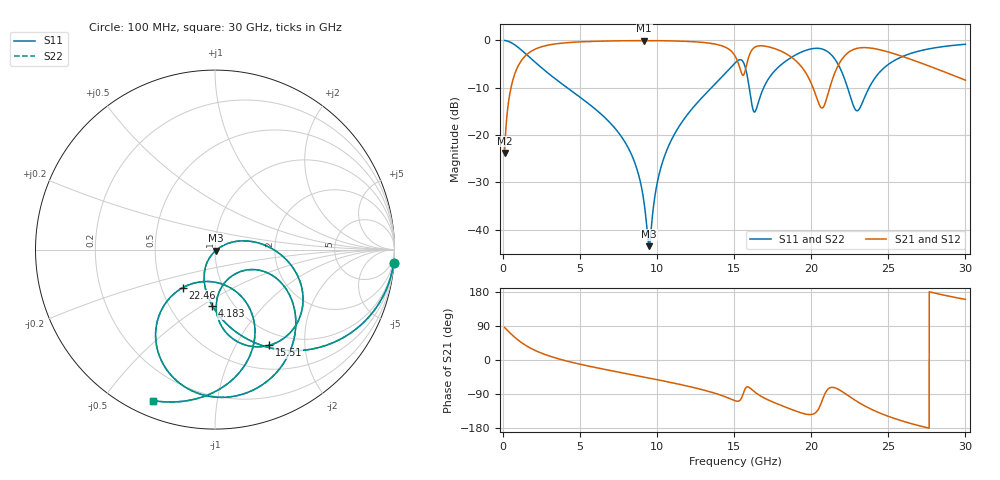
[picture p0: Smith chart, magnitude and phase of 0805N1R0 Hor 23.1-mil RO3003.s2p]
# GHz S MA R 50
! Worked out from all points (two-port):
!   3201 points, 100 MHz to 30 GHz, reference 50 ohm
!   highest |S21| = -0.06 dB at 9.163 GHz (marker M1); lowest = -23.8 dB at 100 MHz (marker M2)
!   |S21| within 3 dB of the highest: 1.516 GHz to 15.01 GHz (13.49 GHz wide, 163 % of centre); 22.23 GHz to 25.6 GHz (3.372 GHz wide, 14.1 % of centre)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
!   lowest |S11| = -43.5 dB at 9.472 GHz (marker M3), VSWR 1.01, Z = 50.4 - j0.519 ohm
!   |S11| at or under -10 dB: 4.151 GHz to 13.53 GHz (9.378 GHz wide, 106 % of centre); 15.97 GHz to 16.91 GHz (937.6 MHz wide, 5.7 % of centre); 22.35 GHz to 23.75 GHz (1.399 GHz wide, 6.07 % of centre)
!   |S22| runs from -43.5 to 0.0 dB; largest |S21 - S12| = 0
!   S11 on the Smith chart (normalised r, x): 100 MHz: 1, -27; 4.183 GHz: 0.80, -0.56; 15.51 GHz: 0.81, -1.39; 22.46 GHz: 0.64, -0.30; 30 GHz: 0.07, -0.67
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0.1  0.9979 -4.2  0.06446 85.8  0.06446 85.8  0.9979 -4.2
0.5017812  0.951 -20.6  0.3086 69.4  0.3086 69.4  0.951 -20.6
1.127813  0.806 -42.1  0.5908 47.9  0.5908 47.9  0.806 -42.1
4.183219  0.3134 -92.7  0.9462 -3.3  0.9462 -3.3  0.3134 -92.7
5.089563  0.244 -101.1  0.9659 -12.0  0.9659 -12.0  0.244 -101.1
7.958094  0.08149 -121.9  0.991 -35.7  0.991 -35.7  0.08149 -121.9
9.163438  0.01855 -115.2  0.9932 -45.2  0.9932 -45.2  0.01855 -115.2
9.471781  0.006665 -50.5  0.993 -47.7  0.993 -47.7  0.006665 -50.5
10.06978  0.03503 25.4  0.9917 -52.5  0.9917 -52.5  0.03503 25.4
13.4055  0.3016 2.6  0.9334 -83.6  0.9334 -83.6  0.3016 2.6
15.05  0.5766 -31.9  0.6847 -107.4  0.6847 -107.4  0.5766 -31.9
15.50784  0.6132 -60.3  0.4381 -97.0  0.4381 -97.0  0.6132 -60.3
15.90028  0.374 -87.8  0.6354 -71.1  0.6354 -71.1  0.374 -87.8
16.33009  0.1749 -53.2  0.8456 -84.3  0.8456 -84.3  0.1749 -53.2
18.22687  0.584 -39.8  0.7429 -122.8  0.7429 -122.8  0.584 -39.8
20.03956  0.8159 -76.9  0.338 -143.6  0.338 -143.6  0.8159 -76.9
20.74969  0.8057 -96.9  0.1943 -102.3  0.1943 -102.3  0.8057 -96.9
21.59997  0.6095 -122.7  0.4841 -74.4  0.4841 -74.4  0.6095 -122.7
22.45959  0.2791 -130.3  0.7565 -95.9  0.7565 -95.9  0.2791 -130.3
23.03891  0.1819 -89.6  0.8278 -111.2  0.8278 -111.2  0.1819 -89.6
25.01978  0.5598 -67.1  0.7518 -149.0  0.7518 -149.0  0.5598 -67.1
30  0.9095 -112.4  0.3796 159.9  0.3796 159.9  0.9095 -112.4
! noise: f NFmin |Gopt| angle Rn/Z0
0.1  0.001459  0.9611  1.299  0.008468
3.417  0.007725  0.7517  18.63  0.006114
6.743  0.01339  0.7249  34.83  0.008821
10.06  0.02022  0.7327  50.42  0.01242
13.39  0.03858  0.8097  65.59  0.03
16.7  0.09567  0.9014  80.68  0.1236
20.03  0.3089  0.9629  94.87  0.8612
23.35  0.1431  0.91  108.5  0.1198
26.67  0.1095  0.8701  121.1  0.0445
30  0.1201  0.8697  133.3  0.03199
